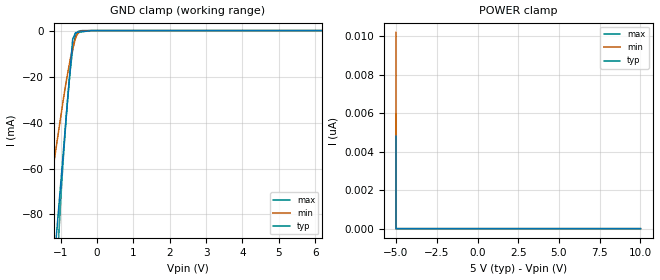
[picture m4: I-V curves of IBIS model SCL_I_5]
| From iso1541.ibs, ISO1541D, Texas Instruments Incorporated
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|   SCL_I Left 5V Input Model
[Model]   SCL_I_5
Model_type   Input
Polarity   Non-Inverting
Enable   Active-Low
Vinl = 0.5
Vinh = 3.85
|   typ   min   max
|   (nom PVT)   (fast PVT)   (slow PVT)
C_comp   3.824p   3.201p   4.341p
|PVT   Nom   Slow   Fast
[Voltage Range]   5   4.5   5.5
[Temperature Range]   27   136   -40
[Power Clamp Reference]   5   4.5   5.5
[GND Clamp Reference]   -0   -0   -0
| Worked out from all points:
|   GND clamp passes 1 mA (typ) near -0.60 V on its own axis
[GND Clamp]
|   Voltage   I(typ)   I(min)   I(max)
-5V       -1.078A    -841.4mA   -1.257A
-1.527V   -179.2mA   -119.4mA   -235.6mA
-1.221V   -108.4mA   -62.47mA   -142.9mA
-1.143V   -93.38mA   -52.43mA   -116.7mA
-1.09V    -83.23mA   -46.82mA   -99.47mA
-1.054V   -76.37mA   -43.03mA   -88.5mA
-929.5mV  -52.67mA   -29.92mA   -55.3mA
-763.8mV  -21.03mA   -14.56mA   -21.24mA
-673.4mV  -3.775mA   -7.956mA   -8.477mA
-606.1mV  -1.346mA   -3.991mA   -2.663mA
-532.7mV  -784.5uA   -1.411mA   -445.1uA
10V       0A         0A         0A
[POWER Clamp]
|   Voltage   I(typ)   I(min)   I(max)
-5V       4.793nA    10.19nA    5.967nA
-5V       0A         0A         0A
-5V       0A         0A         0A
10V       0A         0A         0A
